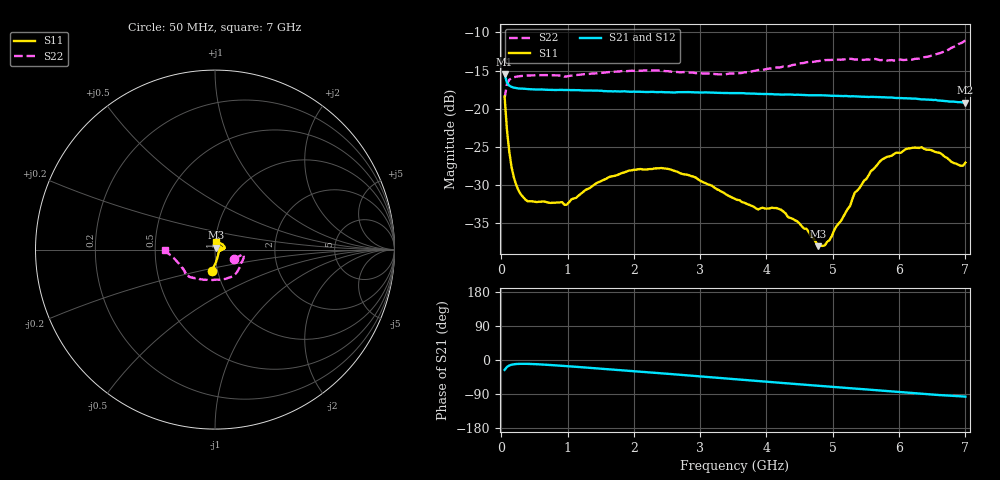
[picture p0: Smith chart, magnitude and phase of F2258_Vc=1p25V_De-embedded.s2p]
! Integrated Device Technology
! Corporate Headquarters
! 6024 Silver Creek Valley Road
! San Jose, CA 95138  USA
! Phone:  1-408-284-8200
! Toll Free:  1-800-223-1366
! Webpage:  http://www.idt.com/
! Timing and RF Division
! 515 Groton Road, Suite 102
! Westford, MA 01886-6024
! Device:  F2258
! Description: Voltage Variable RF Attenuator
! Frequency:  50.0 -  6000.00 MHz
! Package:  3x3 mm Thin QFN Plastic Package: 16 pin
! Ports:  2 RF, 2 DC
!  Pin  1  = NC
!  Pin  2  = NC
!  Pin  3  = RF2  = Port 2
!  Pin  4  = GND
!  Pin  5  = Vdd
!  Pin  6  = NC
!  Pin  7  = VCTRL
!  Pin  8  = NC
!  Pin  9  = GND
!  Pin 10  = RF1  = Port 1
!  Pin 11  = NC
!  Pin 12  = NC
!  Pin 13  = NC
!  Pin 14  = NC
!  Pin 15  = NC
!  Pin 16  = NC
! Vcntrl:  1.250 Volts
! Vdd:  +3.300 Volts
! Current:  1.164 mA
! Data:  The device was measured on a the F2258 evaluation board which has
!  individual transmission lines to the RF pins.  Data was collected
!  using a calibrated network analyzer.  The evaluation board was
!  de-embedded using a TRL calibration technique.
!  The reference plane is the edge of the package pin.
! Misc:  SN 10
!  Action Tracker AT0285
! Date Measured:  2014-12-10
! Date:  2016-01-13  MJV
! Note:
!  Integrated Device Technology supplies this data as a sample of measured
!  data at the package pin for this product.  Your particular data for this
!  product may vary.
!  Data was taken at 25 degrees C.
!  Integrated Device Technology reserves the right to change this data at anytime.
!Freq_(GHz)  S11M_(dB)  S11P_(deg)  S21M_(dB)  S21P_(deg)  S12M_(dB)  S12P_(deg)  S22M_(dB)  S22P_(deg)
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# GHz S dB R 50
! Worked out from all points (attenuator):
!   201 points, 50 MHz to 7 GHz, reference 50 ohm
!   highest |S21| = -15.44 dB at 50 MHz (marker M1); lowest = -19.2 dB at 7 GHz (marker M2)
!   lowest |S11| = -38.0 dB at 4.776 GHz (marker M3), VSWR 1.03, Z = 50.5 + j1.16 ohm
!   |S11| at or under -10 dB: start of sweep to end of sweep
!   |S22| runs from -18.6 to -11.1 dB; largest |S21 - S12| = 0.0012
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0.05  -18.41 -98.2  -15.44 -26.0  -15.44 -26.0  -18.65 -26.9
0.08475  -22.74 -86.6  -16.58 -18.5  -16.58 -18.5  -16.77 -13.3
0.15425  -27.64 -69.4  -17.15 -12.5  -17.15 -12.5  -16.01 -9.7
0.29325  -31.22 -45.2  -17.37 -10.0  -17.36 -10.0  -15.73 -10.6
0.3975  -32.14 -34.7  -17.43 -10.1  -17.45 -10.1  -15.66 -12.5
0.9535  -32.61 -21.5  -17.56 -15.8  -17.54 -15.8  -15.81 -26.3
1.2315  -30.94 -12.7  -17.61 -19.3  -17.61 -19.3  -15.50 -33.3
1.9265  -28.12 0.5  -17.77 -28.5  -17.73 -28.6  -15.06 -48.9
2.37825  -27.81 9.3  -17.83 -34.6  -17.80 -34.6  -15.00 -59.4
2.8995  -28.91 25.6  -17.86 -41.9  -17.92 -41.8  -15.29 -73.6
3.525  -31.83 58.0  -17.96 -50.7  -18.01 -50.6  -15.39 -96.8
3.8725  -33.22 83.0  -18.06 -55.5  -18.09 -55.4  -14.94 -110.0
4.22  -33.25 94.5  -18.16 -60.3  -18.19 -60.2  -14.56 -120.2
4.7065  -36.99 75.3  -18.25 -66.9  -18.28 -66.8  -13.87 -130.2
4.776  -38.02 66.6  -18.25 -67.9  -18.30 -67.8  -13.77 -131.3
4.94975  -37.25 36.1  -18.31 -70.2  -18.36 -70.1  -13.63 -133.5
5.332  -31.01 5.3  -18.39 -75.4  -18.45 -75.3  -13.57 -137.9
5.71425  -26.88 2.6  -18.49 -80.6  -18.53 -80.4  -13.65 -143.5
5.85325  -26.26 4.8  -18.54 -82.4  -18.58 -82.4  -13.66 -146.5
6.33975  -25.05 16.4  -18.78 -89.1  -18.79 -89.1  -13.36 -158.7
6.9305  -27.49 72.7  -19.15 -96.0  -19.20 -95.9  -11.42 -176.7
7  -27.08 85.2  -19.22 -96.6  -19.27 -96.5  -11.06 -179.0
